FUNCTION "Gest Asse Y Foratrice" : VOID
TITLE =Gestione Asse Y Foratrice
AUTHOR : MassimoZ
FAMILY : NovaSrl
VERSION : 0.1

BEGIN
NETWORK
TITLE ======== PACO 1 =======



NETWORK
TITLE =INS./DISIN.1
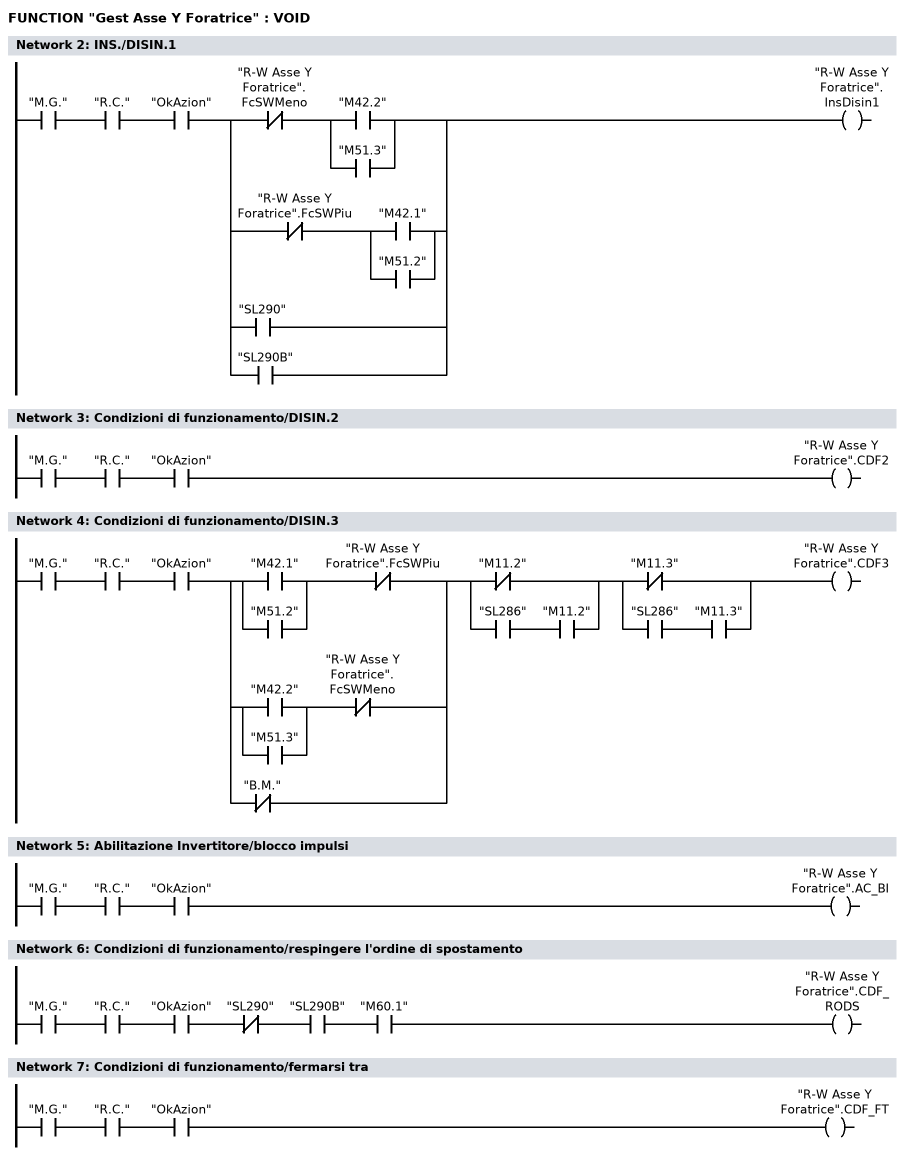
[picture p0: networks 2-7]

      U     "M.G.";
      U     "R.C.";
      U     "OkAzion";
      U(    ;
      UN    "R-W Asse Y Foratrice".FcSWMeno;
      U(    ;
      O     "M42.2";
      O     "M51.3";
      )     ;
      O     ;
      UN    "R-W Asse Y Foratrice".FcSWPiu;
      U(    ;
      O     "M42.1";
      O     "M51.2";
      )     ;
      O     "SL290";
      O     "SL290B";
      )     ;
      =     "R-W Asse Y Foratrice".InsDisin1;
NETWORK
TITLE =Condizioni di funzionamento/DISIN.2

      U     "M.G.";
      U     "R.C.";
      U     "OkAzion";
      =     "R-W Asse Y Foratrice".CDF2;
NETWORK
TITLE =Condizioni di funzionamento/DISIN.3

      U     "M.G.";
      U     "R.C.";
      U     "OkAzion";
      U(    ;
      U(    ;
      O     "M42.1";
      O     "M51.2";
      )     ;
      UN    "R-W Asse Y Foratrice".FcSWPiu;
      O     ;
      U(    ;
      O     "M42.2";
      O     "M51.3";
      )     ;
      UN    "R-W Asse Y Foratrice".FcSWMeno;
      ON    "B.M.";
      )     ;
      U(    ;
      ON    "M11.2";
      O     ;
      U     "SL286";
      U     "M11.2";
      )     ;
      U(    ;
      ON    "M11.3";
      O     ;
      U     "SL286";
      U     "M11.3";
      )     ;
      =     "R-W Asse Y Foratrice".CDF3;
NETWORK
TITLE =Abilitazione Invertitore/blocco impulsi

      U     "M.G.";
      U     "R.C.";
      U     "OkAzion";
      =     "R-W Asse Y Foratrice".AC_BI;
NETWORK
TITLE =Condizioni di funzionamento/respingere l'ordine di spostamento

      U     "M.G.";
      U     "R.C.";
      U     "OkAzion";
      UN    "SL290";
      U     "SL290B";
      U     "M60.1";
      =     "R-W Asse Y Foratrice".CDF_RODS;
NETWORK
TITLE =Condizioni di funzionamento/fermarsi tra

      U     "M.G.";
      U     "R.C.";
      U     "OkAzion";
      =     "R-W Asse Y Foratrice".CDF_FT;
NETWORK
TITLE =Attivare l'oridine di spostamento

      U(    ;
      U(    ;
      O     "M62.0";
      O     "M64.7";
      O     "M66.7";
      O     "M68.7";
      O     "M70.7";
      O     "M72.7";
      O     "M74.7";
      O     "M76.7";
      O     "M64.2";
      O     "M66.2";
      O     "M68.2";
      O     "M70.2";
      O     "M72.2";
      O     "M74.2";
      O     "M76.2";
      )     ;
      UN    "SL290";
      U     "SL290B";
      L     S5T#100MS;
      SE    T     12;
      NOP   0;
      NOP   0;
      NOP   0;
      U     T     12;
      )     ;
      FP    "FronteM251.2";
      =     "R-W Asse Y Foratrice".ALDS;
NETWORK
TITLE =Reset memoria guasti
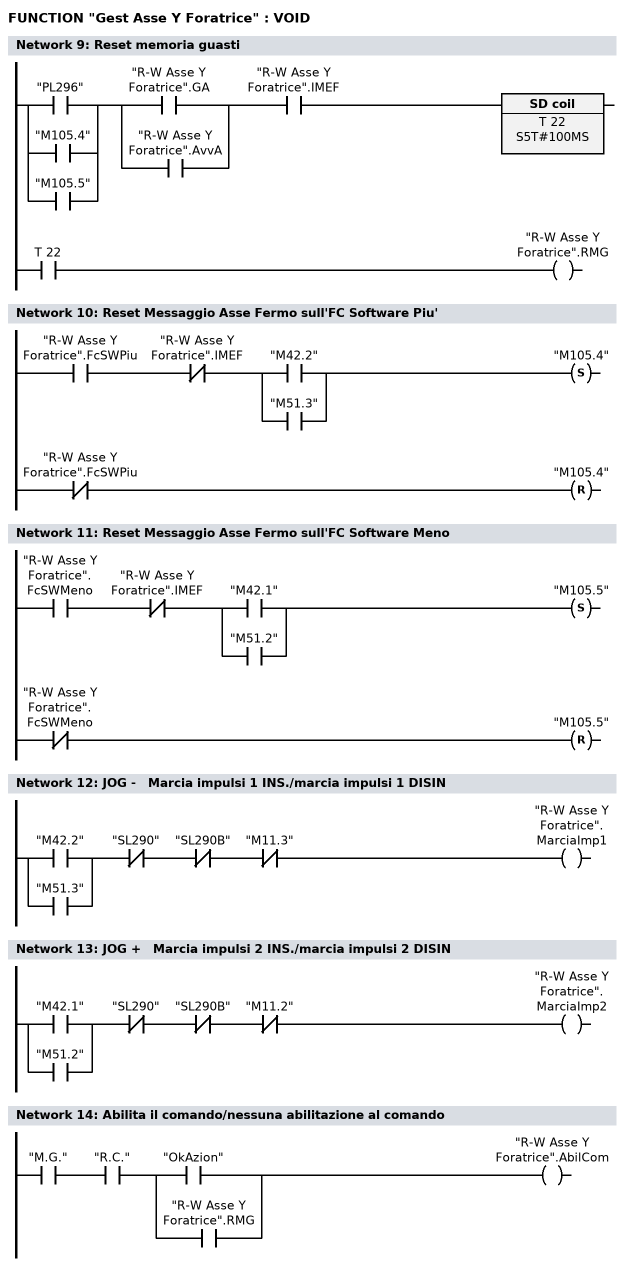
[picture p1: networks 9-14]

      U(    ;
      O     "PL296";
      O     "M105.4";
      O     "M105.5";
      )     ;
      U(    ;
      O     "R-W Asse Y Foratrice".GA;
      O     "R-W Asse Y Foratrice".AvvA;
      )     ;
      U     "R-W Asse Y Foratrice".IMEF;
      L     S5T#100MS;
      SE    T     22;
      NOP   0;
      NOP   0;
      NOP   0;
      U     T     22;
      =     "R-W Asse Y Foratrice".RMG;
NETWORK
TITLE =Reset Messaggio Asse Fermo sull'FC Software Piu'

      U     "R-W Asse Y Foratrice".FcSWPiu;
      UN    "R-W Asse Y Foratrice".IMEF;
      U(    ;
      O     "M42.2";
      O     "M51.3";
      )     ;
      S     "M105.4";
      UN    "R-W Asse Y Foratrice".FcSWPiu;
      R     "M105.4";
      NOP   0;
NETWORK
TITLE =Reset Messaggio Asse Fermo sull'FC Software Meno

      U     "R-W Asse Y Foratrice".FcSWMeno;
      UN    "R-W Asse Y Foratrice".IMEF;
      U(    ;
      O     "M42.1";
      O     "M51.2";
      )     ;
      S     "M105.5";
      UN    "R-W Asse Y Foratrice".FcSWMeno;
      R     "M105.5";
      NOP   0;
NETWORK
TITLE =JOG -   Marcia impulsi 1 INS./marcia impulsi 1 DISIN

      U(    ;
      O     "M42.2";
      O     "M51.3";
      )     ;
      UN    "SL290";
      UN    "SL290B";
      UN    "M11.3";
      =     "R-W Asse Y Foratrice".MarciaImp1;
NETWORK
TITLE =JOG +   Marcia impulsi 2 INS./marcia impulsi 2 DISIN

      U(    ;
      O     "M42.1";
      O     "M51.2";
      )     ;
      UN    "SL290";
      UN    "SL290B";
      UN    "M11.2";
      =     "R-W Asse Y Foratrice".MarciaImp2;
NETWORK
TITLE =Abilita il comando/nessuna abilitazione al comando

      U     "M.G.";
      U     "R.C.";
      U(    ;
      O     "OkAzion";
      O     "R-W Asse Y Foratrice".RMG;
      )     ;
      =     "R-W Asse Y Foratrice".AbilCom;
NETWORK
TITLE =Com Aut Apertura Pinza Foratrice per Ref Point

      U(    ;
      U     "SL290";
      UN    "SL290B";
      U     "PL292";
      S     "M105.6";
      U(    ;
      ON    "M.G.";
      ON    "SL290";
      O     "M11.2";
      O     "M11.3";
      )     ;
      R     "M105.6";
      U     "M105.6";
      )     ;
      L     "Scambio dati OP".TempApePinzaFor;
      SE    "T6";
      NOP   0;
      NOP   0;
      NOP   0;
      NOP   0;
NETWORK
TITLE =Avvio a riferirsi/interruzione del riferirsi
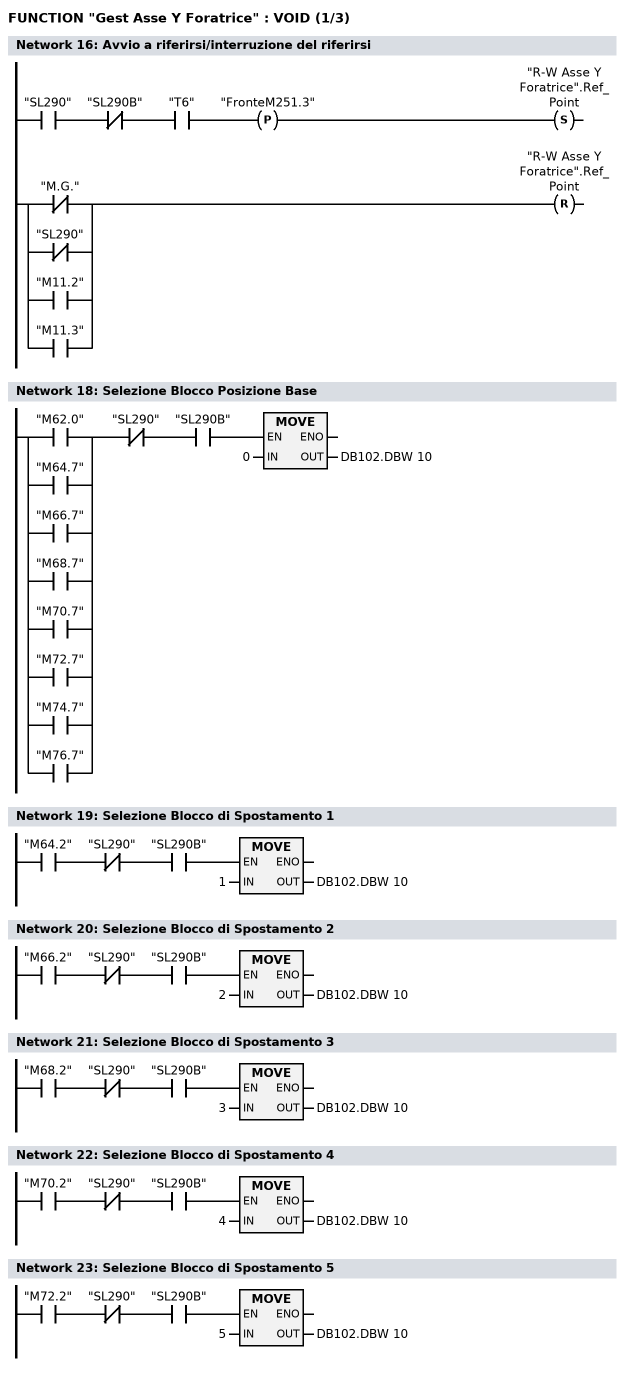
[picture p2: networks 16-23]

      U     "SL290";
      UN    "SL290B";
      U     "T6";
      FP    "FronteM251.3";
      S     "R-W Asse Y Foratrice".Ref_Point;
      U(    ;
      ON    "M.G.";
      ON    "SL290";
      O     "M11.2";
      O     "M11.3";
      )     ;
      R     "R-W Asse Y Foratrice".Ref_Point;
      NOP   0;
NETWORK
TITLE ======== SCELTA BLOCCO =======

NETWORK
TITLE =Selezione Blocco Posizione Base

      U(    ;
      O     "M62.0";
      O     "M64.7";
      O     "M66.7";
      O     "M68.7";
      O     "M70.7";
      O     "M72.7";
      O     "M74.7";
      O     "M76.7";
      )     ;
      UN    "SL290";
      U     "SL290B";
      SPBNB _001;
      L     0;
      T     DB102.DBW   10;
_001: NOP   0;
NETWORK
TITLE =Selezione Blocco di Spostamento 1

      U     "M64.2";
      UN    "SL290";
      U     "SL290B";
      SPBNB _002;
      L     1;
      T     DB102.DBW   10;
_002: NOP   0;
NETWORK
TITLE =Selezione Blocco di Spostamento 2

      U     "M66.2";
      UN    "SL290";
      U     "SL290B";
      SPBNB _003;
      L     2;
      T     DB102.DBW   10;
_003: NOP   0;
NETWORK
TITLE =Selezione Blocco di Spostamento 3

      U     "M68.2";
      UN    "SL290";
      U     "SL290B";
      SPBNB _004;
      L     3;
      T     DB102.DBW   10;
_004: NOP   0;
NETWORK
TITLE =Selezione Blocco di Spostamento 4

      U     "M70.2";
      UN    "SL290";
      U     "SL290B";
      SPBNB _005;
      L     4;
      T     DB102.DBW   10;
_005: NOP   0;
NETWORK
TITLE =Selezione Blocco di Spostamento 5

      U     "M72.2";
      UN    "SL290";
      U     "SL290B";
      SPBNB _006;
      L     5;
      T     DB102.DBW   10;
_006: NOP   0;
NETWORK
TITLE =Selezione Blocco di Spostamento 6
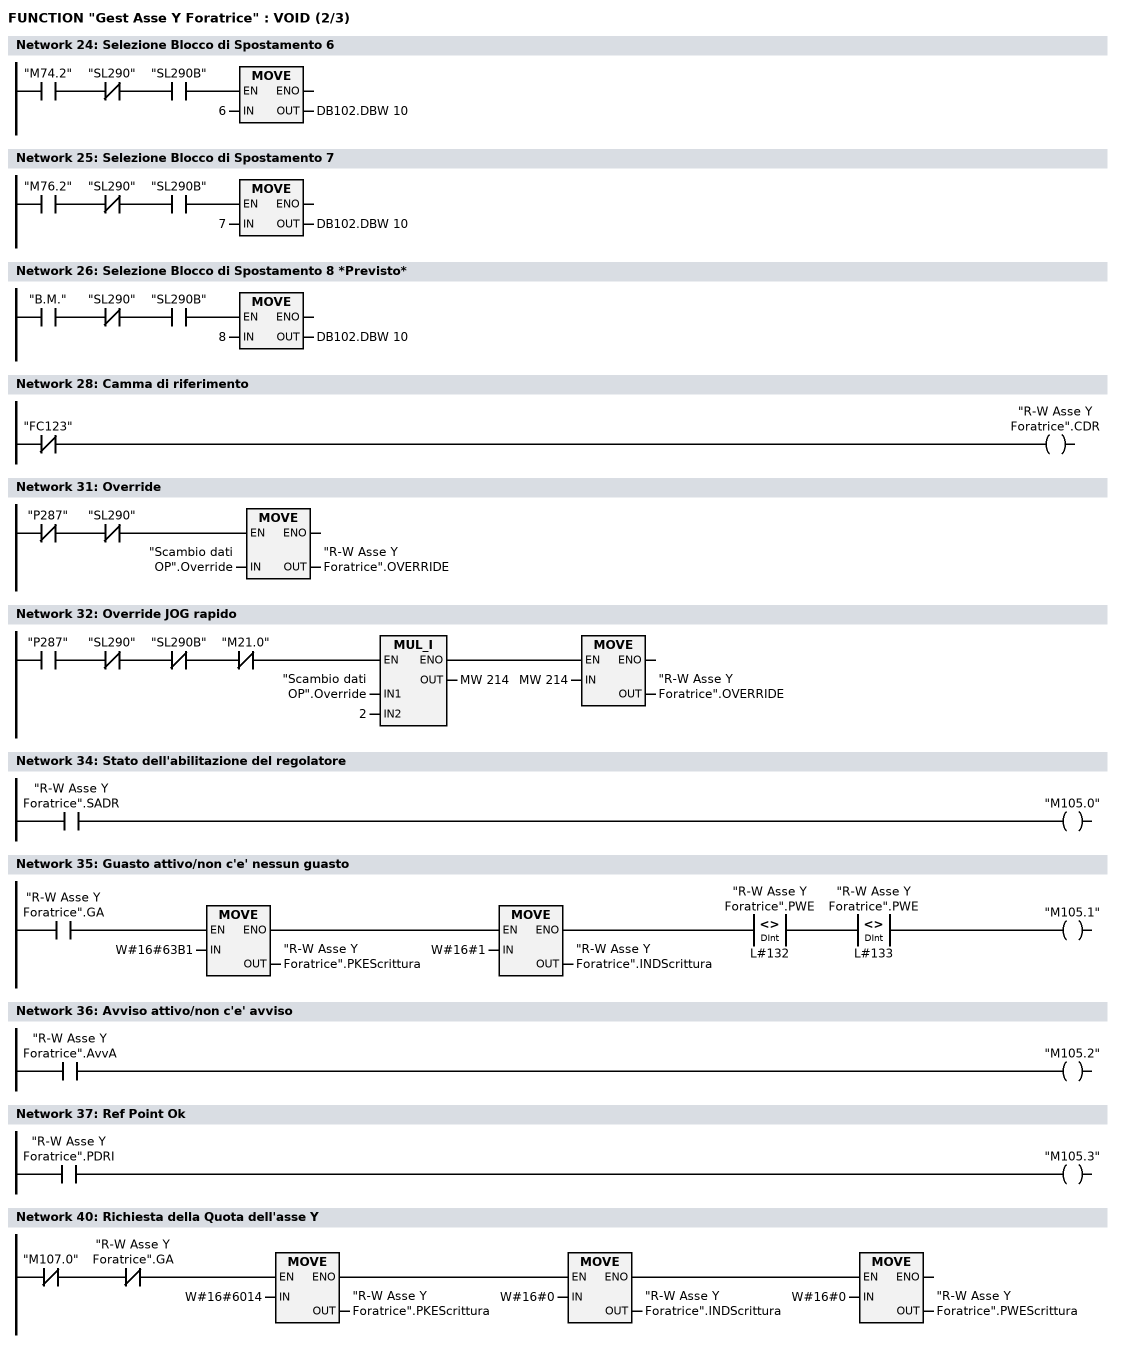
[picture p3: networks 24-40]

      U     "M74.2";
      UN    "SL290";
      U     "SL290B";
      SPBNB _007;
      L     6;
      T     DB102.DBW   10;
_007: NOP   0;
NETWORK
TITLE =Selezione Blocco di Spostamento 7

      U     "M76.2";
      UN    "SL290";
      U     "SL290B";
      SPBNB _008;
      L     7;
      T     DB102.DBW   10;
_008: NOP   0;
NETWORK
TITLE =Selezione Blocco di Spostamento 8 *Previsto*

      U     "B.M.";
      UN    "SL290";
      U     "SL290B";
      SPBNB _009;
      L     8;
      T     DB102.DBW   10;
_009: NOP   0;
NETWORK
TITLE ======== POS PACO =======



NETWORK
TITLE =Camma di riferimento

      UN    "FC123";
      =     "R-W Asse Y Foratrice".CDR;
NETWORK
TITLE ======== PACO 2 ======= ( previsto )



NETWORK
TITLE ======== OVERRIDE ======



NETWORK
TITLE =Override

      UN    "P287";
      UN    "SL290";
      SPBNB _00a;
      L     "Scambio dati OP".Override;
      T     "R-W Asse Y Foratrice".OVERRIDE;
_00a: NOP   0;
NETWORK
TITLE =Override JOG rapido

      U(    ;
      U     "P287";
      UN    "SL290";
      UN    "SL290B";
      UN    "M21.0";
      SPBNB _00b;
      L     "Scambio dati OP".Override;
      L     2;
      *I    ;
      T     MW   214;
      UN    OV;
      SAVE  ;
      CLR   ;
_00b: U     BIE;
      )     ;
      SPBNB _00c;
      L     MW   214;
      T     "R-W Asse Y Foratrice".OVERRIDE;
_00c: NOP   0;
NETWORK
TITLE ======== PAST 1 =======



NETWORK
TITLE =Stato dell'abilitazione del regolatore

      U     "R-W Asse Y Foratrice".SADR;
      =     "M105.0";
NETWORK
TITLE =Guasto attivo/non c'e' nessun guasto

      U(    ;
      U(    ;
      U     "R-W Asse Y Foratrice".GA;
      SPBNB _00d;
      L     W#16#63B1;
      T     "R-W Asse Y Foratrice".PKEScrittura;
      SET   ;
      SAVE  ;
      CLR   ;
_00d: U     BIE;
      )     ;
      SPBNB _00e;
      L     W#16#1;
      T     "R-W Asse Y Foratrice".INDScrittura;
      SET   ;
      SAVE  ;
      CLR   ;
_00e: U     BIE;
      )     ;
      U(    ;
      L     "R-W Asse Y Foratrice".PWE;
      L     L#132;
      <>D   ;
      )     ;
      U(    ;
      L     "R-W Asse Y Foratrice".PWE;
      L     L#133;
      <>D   ;
      )     ;
      =     "M105.1";
NETWORK
TITLE =Avviso attivo/non c'e' avviso

      U     "R-W Asse Y Foratrice".AvvA;
      =     "M105.2";
NETWORK
TITLE =Ref Point Ok

      U     "R-W Asse Y Foratrice".PDRI;
      =     "M105.3";
NETWORK
TITLE ======== POS PAST =======



NETWORK
TITLE ======== Lettura Quote =======



NETWORK
TITLE =Richiesta della Quota dell'asse Y

      U(    ;
      U(    ;
      UN    "M107.0";
      UN    "R-W Asse Y Foratrice".GA;
      SPBNB _00f;
      L     W#16#6014;
      T     "R-W Asse Y Foratrice".PKEScrittura;
      SET   ;
      SAVE  ;
      CLR   ;
_00f: U     BIE;
      )     ;
      SPBNB _010;
      L     W#16#0;
      T     "R-W Asse Y Foratrice".INDScrittura;
      SET   ;
      SAVE  ;
      CLR   ;
_010: U     BIE;
      )     ;
      SPBNB _011;
      L     W#16#0;
      T     "R-W Asse Y Foratrice".PWEScrittura;
_011: NOP   0;
NETWORK
TITLE =Lettura Quota Asse Y
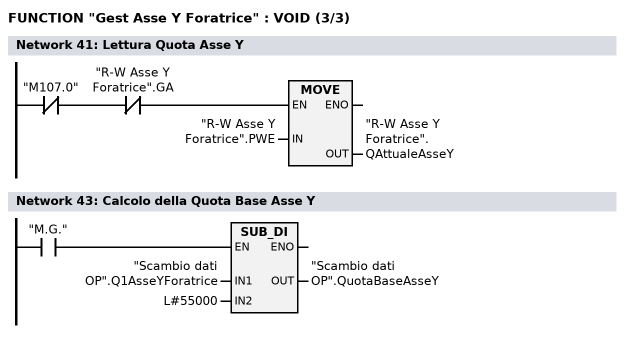
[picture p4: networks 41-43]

      UN    "M107.0";
      UN    "R-W Asse Y Foratrice".GA;
      SPBNB _012;
      L     "R-W Asse Y Foratrice".PWE;
      T     "R-W Asse Y Foratrice".QAttualeAsseY;
_012: NOP   0;
NETWORK
TITLE ======== Caricamento quote sui Blocchi di Spostamento =======



NETWORK
TITLE =Calcolo della Quota Base Asse Y

      U     "M.G.";
      SPBNB _013;
      L     "Scambio dati OP".Q1AsseYForatrice;
      L     L#55000;
      -D    ;
      T     "Scambio dati OP".QuotaBaseAsseY;
_013: NOP   0;
NETWORK
TITLE =Caricamento Primo Posizionamento

      UN    "SL290";
      UN    "SL290B";
      U     "Area Interfaccia OP  PLC".TDT;
      O     "M107.0";
      O(    ;
      U     "M.G.";
      FP    "FronteM252.6";
      )     ;
      =     L      0.0;
      U(    ;
      U(    ;
      U     L      0.0;
      UN    M    107.1;
      SPBNB _014;
      L     W#16#8051;
      T     "R-W Asse Y Foratrice".PKEScrittura;
      SET   ;
      SAVE  ;
      CLR   ;
_014: U     BIE;
      )     ;
      SPBNB _015;
      L     W#16#1;
      T     "R-W Asse Y Foratrice".INDScrittura;
      SET   ;
      SAVE  ;
      CLR   ;
_015: U     BIE;
      )     ;
      SPBNB _016;
      L     "Scambio dati OP".Q1AsseYForatrice;
      T     "R-W Asse Y Foratrice".PWEScrittura;
_016: NOP   0;
      U     L      0.0;
      BLD   102;
      S     "M107.0";
NETWORK
TITLE =Confronto Primo Posizionamento caricato nel 611U
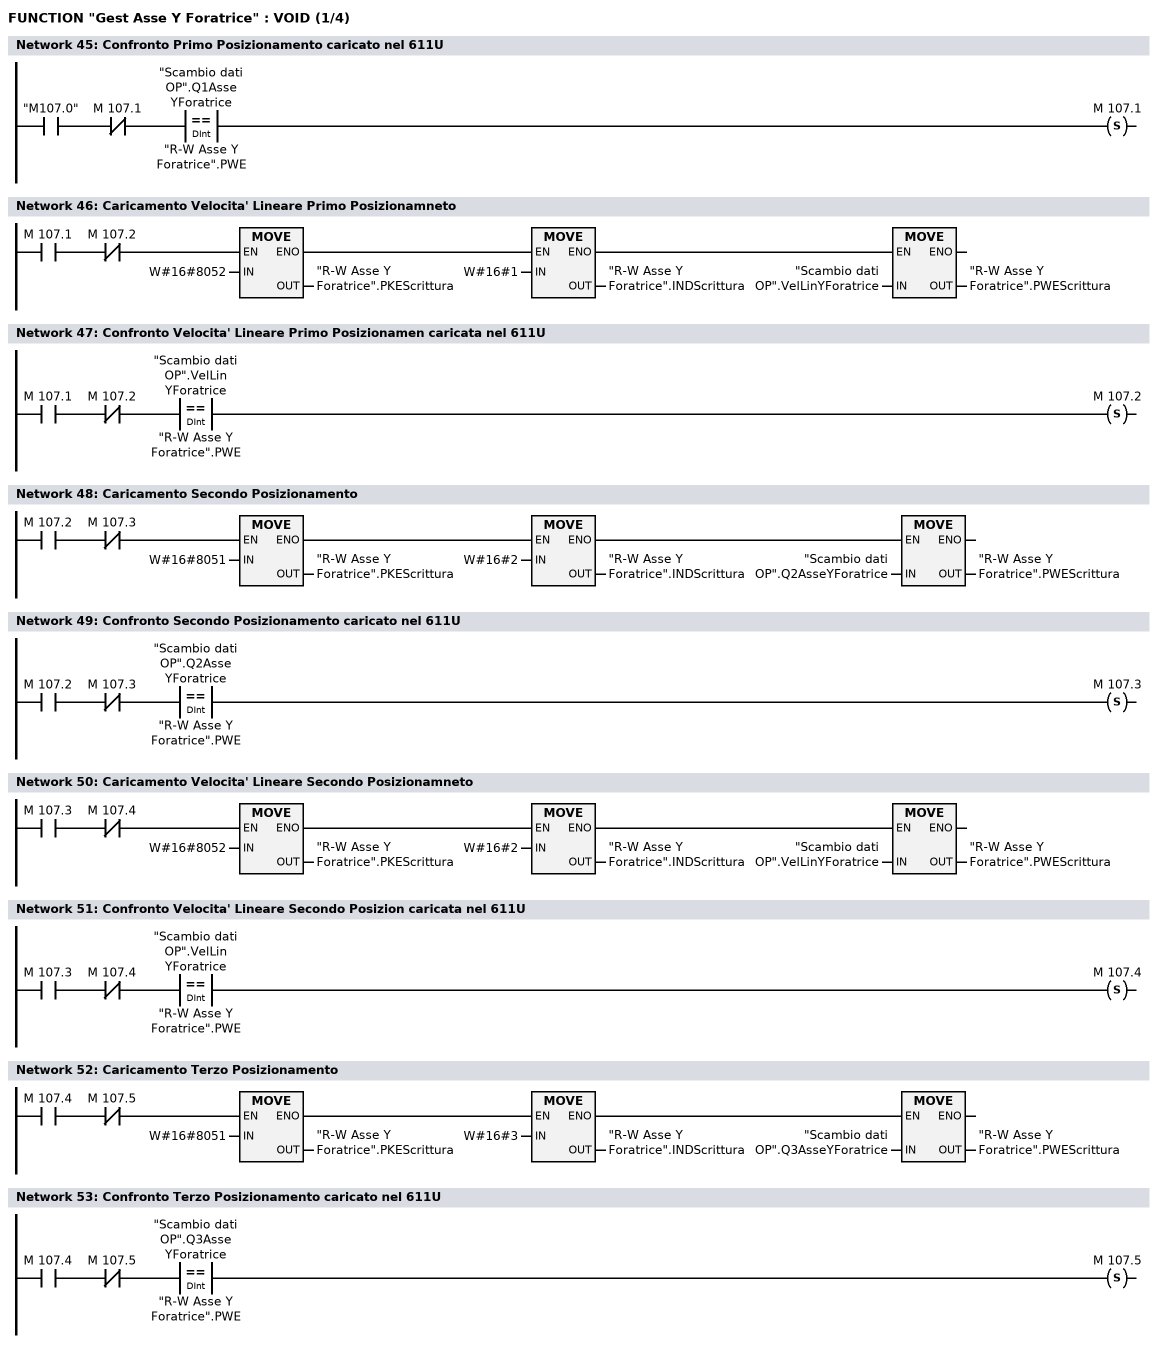
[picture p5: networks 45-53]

      U     "M107.0";
      UN    M    107.1;
      U(    ;
      L     "Scambio dati OP".Q1AsseYForatrice;
      L     "R-W Asse Y Foratrice".PWE;
      ==D   ;
      )     ;
      S     M    107.1;
NETWORK
TITLE =Caricamento Velocita' Lineare Primo Posizionamneto

      U(    ;
      U(    ;
      U     M    107.1;
      UN    M    107.2;
      SPBNB _017;
      L     W#16#8052;
      T     "R-W Asse Y Foratrice".PKEScrittura;
      SET   ;
      SAVE  ;
      CLR   ;
_017: U     BIE;
      )     ;
      SPBNB _018;
      L     W#16#1;
      T     "R-W Asse Y Foratrice".INDScrittura;
      SET   ;
      SAVE  ;
      CLR   ;
_018: U     BIE;
      )     ;
      SPBNB _019;
      L     "Scambio dati OP".VelLinYForatrice;
      T     "R-W Asse Y Foratrice".PWEScrittura;
_019: NOP   0;
NETWORK
TITLE =Confronto Velocita' Lineare Primo Posizionamen caricata nel 611U

      U     M    107.1;
      UN    M    107.2;
      U(    ;
      L     "Scambio dati OP".VelLinYForatrice;
      L     "R-W Asse Y Foratrice".PWE;
      ==D   ;
      )     ;
      S     M    107.2;
NETWORK
TITLE =Caricamento Secondo Posizionamento

      U(    ;
      U(    ;
      U     M    107.2;
      UN    M    107.3;
      SPBNB _01a;
      L     W#16#8051;
      T     "R-W Asse Y Foratrice".PKEScrittura;
      SET   ;
      SAVE  ;
      CLR   ;
_01a: U     BIE;
      )     ;
      SPBNB _01b;
      L     W#16#2;
      T     "R-W Asse Y Foratrice".INDScrittura;
      SET   ;
      SAVE  ;
      CLR   ;
_01b: U     BIE;
      )     ;
      SPBNB _01c;
      L     "Scambio dati OP".Q2AsseYForatrice;
      T     "R-W Asse Y Foratrice".PWEScrittura;
_01c: NOP   0;
NETWORK
TITLE =Confronto Secondo Posizionamento caricato nel 611U

      U     M    107.2;
      UN    M    107.3;
      U(    ;
      L     "Scambio dati OP".Q2AsseYForatrice;
      L     "R-W Asse Y Foratrice".PWE;
      ==D   ;
      )     ;
      S     M    107.3;
NETWORK
TITLE =Caricamento Velocita' Lineare Secondo Posizionamneto

      U(    ;
      U(    ;
      U     M    107.3;
      UN    M    107.4;
      SPBNB _01d;
      L     W#16#8052;
      T     "R-W Asse Y Foratrice".PKEScrittura;
      SET   ;
      SAVE  ;
      CLR   ;
_01d: U     BIE;
      )     ;
      SPBNB _01e;
      L     W#16#2;
      T     "R-W Asse Y Foratrice".INDScrittura;
      SET   ;
      SAVE  ;
      CLR   ;
_01e: U     BIE;
      )     ;
      SPBNB _01f;
      L     "Scambio dati OP".VelLinYForatrice;
      T     "R-W Asse Y Foratrice".PWEScrittura;
_01f: NOP   0;
NETWORK
TITLE =Confronto Velocita' Lineare Secondo Posizion caricata nel 611U

      U     M    107.3;
      UN    M    107.4;
      U(    ;
      L     "Scambio dati OP".VelLinYForatrice;
      L     "R-W Asse Y Foratrice".PWE;
      ==D   ;
      )     ;
      S     M    107.4;
NETWORK
TITLE =Caricamento Terzo Posizionamento

      U(    ;
      U(    ;
      U     M    107.4;
      UN    M    107.5;
      SPBNB _020;
      L     W#16#8051;
      T     "R-W Asse Y Foratrice".PKEScrittura;
      SET   ;
      SAVE  ;
      CLR   ;
_020: U     BIE;
      )     ;
      SPBNB _021;
      L     W#16#3;
      T     "R-W Asse Y Foratrice".INDScrittura;
      SET   ;
      SAVE  ;
      CLR   ;
_021: U     BIE;
      )     ;
      SPBNB _022;
      L     "Scambio dati OP".Q3AsseYForatrice;
      T     "R-W Asse Y Foratrice".PWEScrittura;
_022: NOP   0;
NETWORK
TITLE =Confronto Terzo Posizionamento caricato nel 611U

      U     M    107.4;
      UN    M    107.5;
      U(    ;
      L     "Scambio dati OP".Q3AsseYForatrice;
      L     "R-W Asse Y Foratrice".PWE;
      ==D   ;
      )     ;
      S     M    107.5;
NETWORK
TITLE =Caricamento Velocita' Lineare Terzo Posizionamento
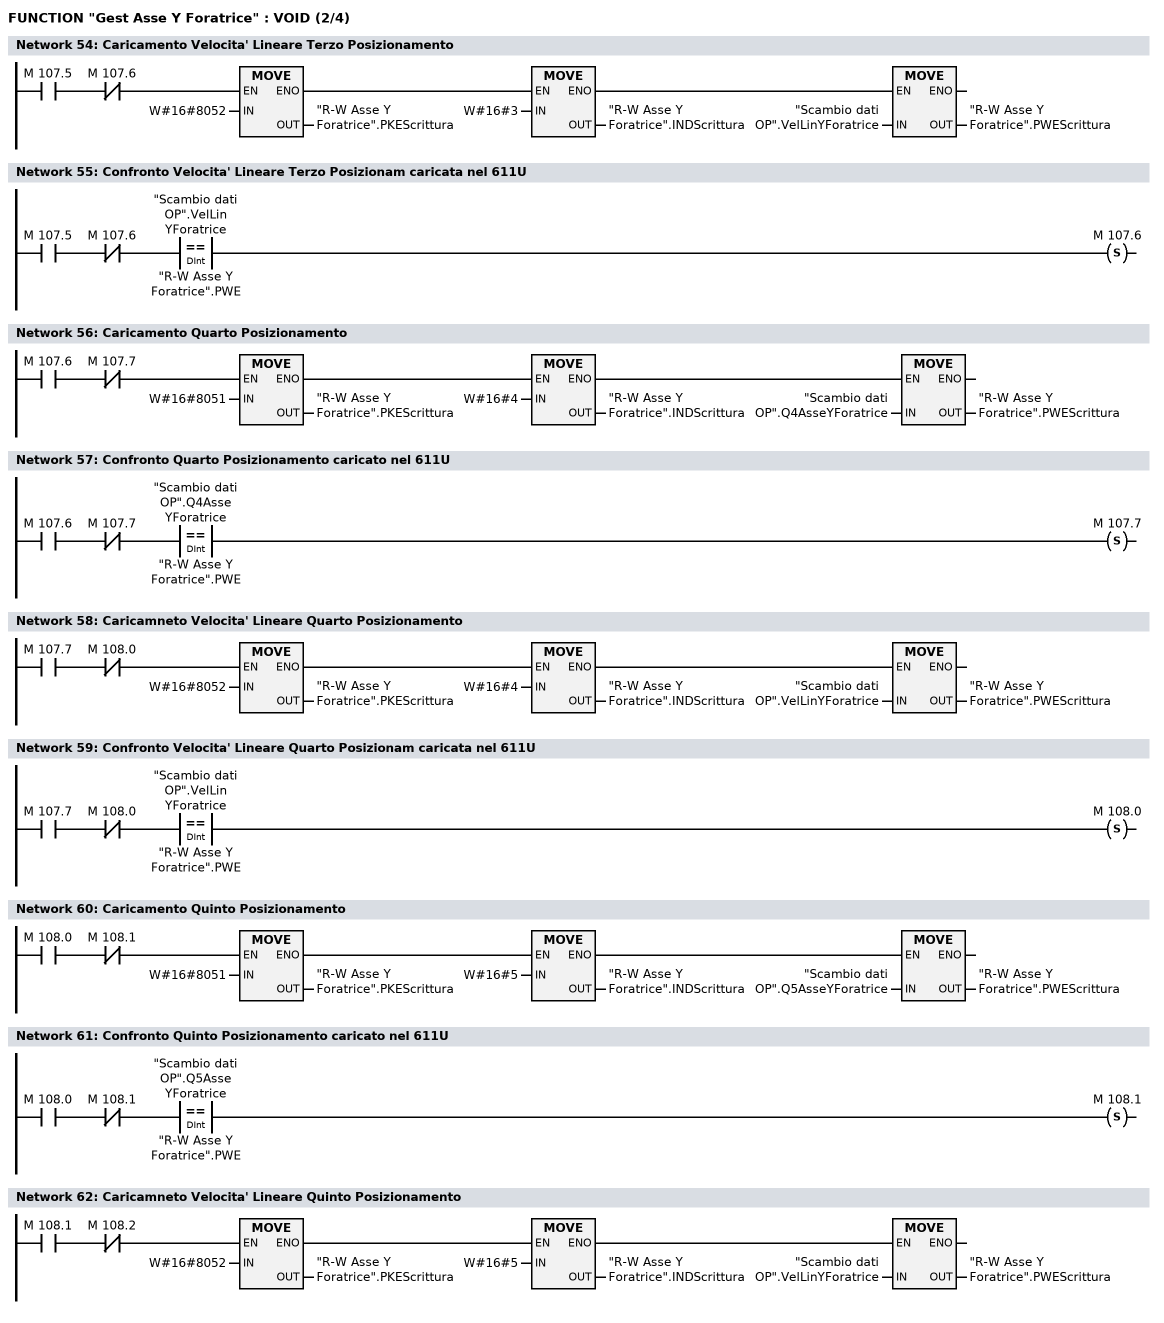
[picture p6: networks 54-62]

      U(    ;
      U(    ;
      U     M    107.5;
      UN    M    107.6;
      SPBNB _023;
      L     W#16#8052;
      T     "R-W Asse Y Foratrice".PKEScrittura;
      SET   ;
      SAVE  ;
      CLR   ;
_023: U     BIE;
      )     ;
      SPBNB _024;
      L     W#16#3;
      T     "R-W Asse Y Foratrice".INDScrittura;
      SET   ;
      SAVE  ;
      CLR   ;
_024: U     BIE;
      )     ;
      SPBNB _025;
      L     "Scambio dati OP".VelLinYForatrice;
      T     "R-W Asse Y Foratrice".PWEScrittura;
_025: NOP   0;
NETWORK
TITLE =Confronto Velocita' Lineare Terzo Posizionam caricata nel 611U

      U     M    107.5;
      UN    M    107.6;
      U(    ;
      L     "Scambio dati OP".VelLinYForatrice;
      L     "R-W Asse Y Foratrice".PWE;
      ==D   ;
      )     ;
      S     M    107.6;
NETWORK
TITLE =Caricamento Quarto Posizionamento

      U(    ;
      U(    ;
      U     M    107.6;
      UN    M    107.7;
      SPBNB _026;
      L     W#16#8051;
      T     "R-W Asse Y Foratrice".PKEScrittura;
      SET   ;
      SAVE  ;
      CLR   ;
_026: U     BIE;
      )     ;
      SPBNB _027;
      L     W#16#4;
      T     "R-W Asse Y Foratrice".INDScrittura;
      SET   ;
      SAVE  ;
      CLR   ;
_027: U     BIE;
      )     ;
      SPBNB _028;
      L     "Scambio dati OP".Q4AsseYForatrice;
      T     "R-W Asse Y Foratrice".PWEScrittura;
_028: NOP   0;
NETWORK
TITLE =Confronto Quarto Posizionamento caricato nel 611U

      U     M    107.6;
      UN    M    107.7;
      U(    ;
      L     "Scambio dati OP".Q4AsseYForatrice;
      L     "R-W Asse Y Foratrice".PWE;
      ==D   ;
      )     ;
      S     M    107.7;
NETWORK
TITLE =Caricamneto Velocita' Lineare Quarto Posizionamento

      U(    ;
      U(    ;
      U     M    107.7;
      UN    M    108.0;
      SPBNB _029;
      L     W#16#8052;
      T     "R-W Asse Y Foratrice".PKEScrittura;
      SET   ;
      SAVE  ;
      CLR   ;
_029: U     BIE;
      )     ;
      SPBNB _02a;
      L     W#16#4;
      T     "R-W Asse Y Foratrice".INDScrittura;
      SET   ;
      SAVE  ;
      CLR   ;
_02a: U     BIE;
      )     ;
      SPBNB _02b;
      L     "Scambio dati OP".VelLinYForatrice;
      T     "R-W Asse Y Foratrice".PWEScrittura;
_02b: NOP   0;
NETWORK
TITLE =Confronto Velocita' Lineare Quarto Posizionam caricata nel 611U

      U     M    107.7;
      UN    M    108.0;
      U(    ;
      L     "Scambio dati OP".VelLinYForatrice;
      L     "R-W Asse Y Foratrice".PWE;
      ==D   ;
      )     ;
      S     M    108.0;
NETWORK
TITLE =Caricamento Quinto Posizionamento

      U(    ;
      U(    ;
      U     M    108.0;
      UN    M    108.1;
      SPBNB _02c;
      L     W#16#8051;
      T     "R-W Asse Y Foratrice".PKEScrittura;
      SET   ;
      SAVE  ;
      CLR   ;
_02c: U     BIE;
      )     ;
      SPBNB _02d;
      L     W#16#5;
      T     "R-W Asse Y Foratrice".INDScrittura;
      SET   ;
      SAVE  ;
      CLR   ;
_02d: U     BIE;
      )     ;
      SPBNB _02e;
      L     "Scambio dati OP".Q5AsseYForatrice;
      T     "R-W Asse Y Foratrice".PWEScrittura;
_02e: NOP   0;
NETWORK
TITLE =Confronto Quinto Posizionamento caricato nel 611U

      U     M    108.0;
      UN    M    108.1;
      U(    ;
      L     "Scambio dati OP".Q5AsseYForatrice;
      L     "R-W Asse Y Foratrice".PWE;
      ==D   ;
      )     ;
      S     M    108.1;
NETWORK
TITLE =Caricamneto Velocita' Lineare Quinto Posizionamento

      U(    ;
      U(    ;
      U     M    108.1;
      UN    M    108.2;
      SPBNB _02f;
      L     W#16#8052;
      T     "R-W Asse Y Foratrice".PKEScrittura;
      SET   ;
      SAVE  ;
      CLR   ;
_02f: U     BIE;
      )     ;
      SPBNB _030;
      L     W#16#5;
      T     "R-W Asse Y Foratrice".INDScrittura;
      SET   ;
      SAVE  ;
      CLR   ;
_030: U     BIE;
      )     ;
      SPBNB _031;
      L     "Scambio dati OP".VelLinYForatrice;
      T     "R-W Asse Y Foratrice".PWEScrittura;
_031: NOP   0;
NETWORK
TITLE =Confronto Velocita' Lineare Quinto Posizionam caricata nel 611U
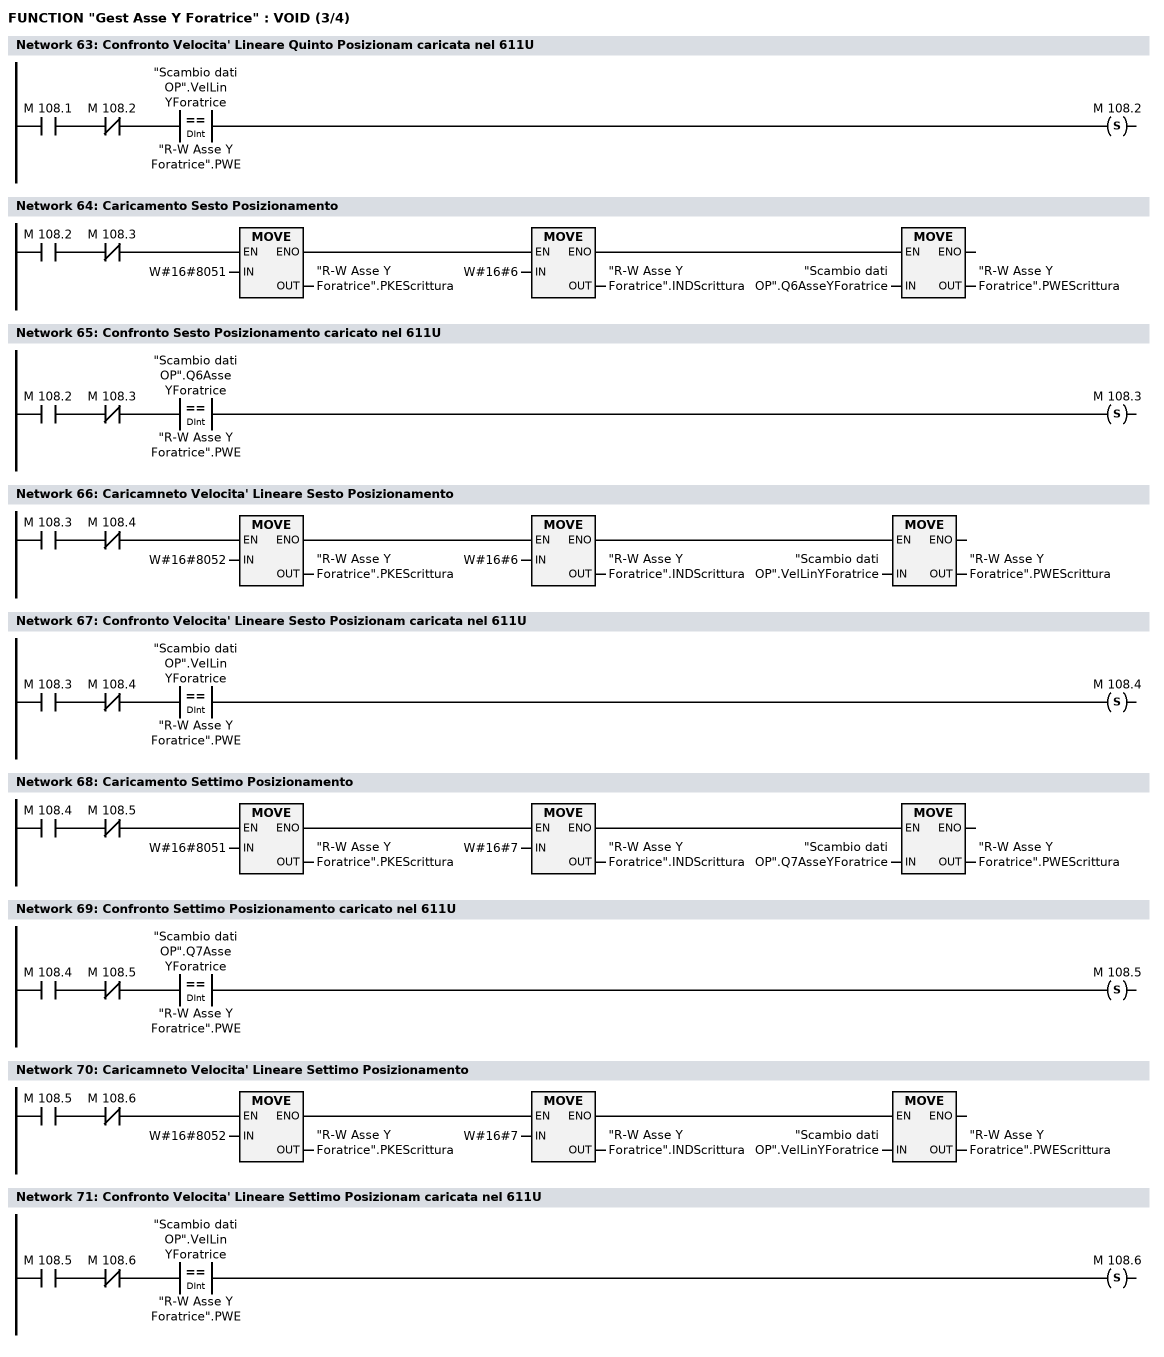
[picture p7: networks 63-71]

      U     M    108.1;
      UN    M    108.2;
      U(    ;
      L     "Scambio dati OP".VelLinYForatrice;
      L     "R-W Asse Y Foratrice".PWE;
      ==D   ;
      )     ;
      S     M    108.2;
NETWORK
TITLE =Caricamento Sesto Posizionamento

      U(    ;
      U(    ;
      U     M    108.2;
      UN    M    108.3;
      SPBNB _032;
      L     W#16#8051;
      T     "R-W Asse Y Foratrice".PKEScrittura;
      SET   ;
      SAVE  ;
      CLR   ;
_032: U     BIE;
      )     ;
      SPBNB _033;
      L     W#16#6;
      T     "R-W Asse Y Foratrice".INDScrittura;
      SET   ;
      SAVE  ;
      CLR   ;
_033: U     BIE;
      )     ;
      SPBNB _034;
      L     "Scambio dati OP".Q6AsseYForatrice;
      T     "R-W Asse Y Foratrice".PWEScrittura;
_034: NOP   0;
NETWORK
TITLE =Confronto Sesto Posizionamento caricato nel 611U

      U     M    108.2;
      UN    M    108.3;
      U(    ;
      L     "Scambio dati OP".Q6AsseYForatrice;
      L     "R-W Asse Y Foratrice".PWE;
      ==D   ;
      )     ;
      S     M    108.3;
NETWORK
TITLE =Caricamneto Velocita' Lineare Sesto Posizionamento

      U(    ;
      U(    ;
      U     M    108.3;
      UN    M    108.4;
      SPBNB _035;
      L     W#16#8052;
      T     "R-W Asse Y Foratrice".PKEScrittura;
      SET   ;
      SAVE  ;
      CLR   ;
_035: U     BIE;
      )     ;
      SPBNB _036;
      L     W#16#6;
      T     "R-W Asse Y Foratrice".INDScrittura;
      SET   ;
      SAVE  ;
      CLR   ;
_036: U     BIE;
      )     ;
      SPBNB _037;
      L     "Scambio dati OP".VelLinYForatrice;
      T     "R-W Asse Y Foratrice".PWEScrittura;
_037: NOP   0;
NETWORK
TITLE =Confronto Velocita' Lineare Sesto Posizionam caricata nel 611U

      U     M    108.3;
      UN    M    108.4;
      U(    ;
      L     "Scambio dati OP".VelLinYForatrice;
      L     "R-W Asse Y Foratrice".PWE;
      ==D   ;
      )     ;
      S     M    108.4;
NETWORK
TITLE =Caricamento Settimo Posizionamento

      U(    ;
      U(    ;
      U     M    108.4;
      UN    M    108.5;
      SPBNB _038;
      L     W#16#8051;
      T     "R-W Asse Y Foratrice".PKEScrittura;
      SET   ;
      SAVE  ;
      CLR   ;
_038: U     BIE;
      )     ;
      SPBNB _039;
      L     W#16#7;
      T     "R-W Asse Y Foratrice".INDScrittura;
      SET   ;
      SAVE  ;
      CLR   ;
_039: U     BIE;
      )     ;
      SPBNB _03a;
      L     "Scambio dati OP".Q7AsseYForatrice;
      T     "R-W Asse Y Foratrice".PWEScrittura;
_03a: NOP   0;
NETWORK
TITLE =Confronto Settimo Posizionamento caricato nel 611U

      U     M    108.4;
      UN    M    108.5;
      U(    ;
      L     "Scambio dati OP".Q7AsseYForatrice;
      L     "R-W Asse Y Foratrice".PWE;
      ==D   ;
      )     ;
      S     M    108.5;
NETWORK
TITLE =Caricamneto Velocita' Lineare Settimo Posizionamento

      U(    ;
      U(    ;
      U     M    108.5;
      UN    M    108.6;
      SPBNB _03b;
      L     W#16#8052;
      T     "R-W Asse Y Foratrice".PKEScrittura;
      SET   ;
      SAVE  ;
      CLR   ;
_03b: U     BIE;
      )     ;
      SPBNB _03c;
      L     W#16#7;
      T     "R-W Asse Y Foratrice".INDScrittura;
      SET   ;
      SAVE  ;
      CLR   ;
_03c: U     BIE;
      )     ;
      SPBNB _03d;
      L     "Scambio dati OP".VelLinYForatrice;
      T     "R-W Asse Y Foratrice".PWEScrittura;
_03d: NOP   0;
NETWORK
TITLE =Confronto Velocita' Lineare Settimo Posizionam caricata nel 611U

      U     M    108.5;
      UN    M    108.6;
      U(    ;
      L     "Scambio dati OP".VelLinYForatrice;
      L     "R-W Asse Y Foratrice".PWE;
      ==D   ;
      )     ;
      S     M    108.6;
NETWORK
TITLE =Caricamento Posizionamento Base
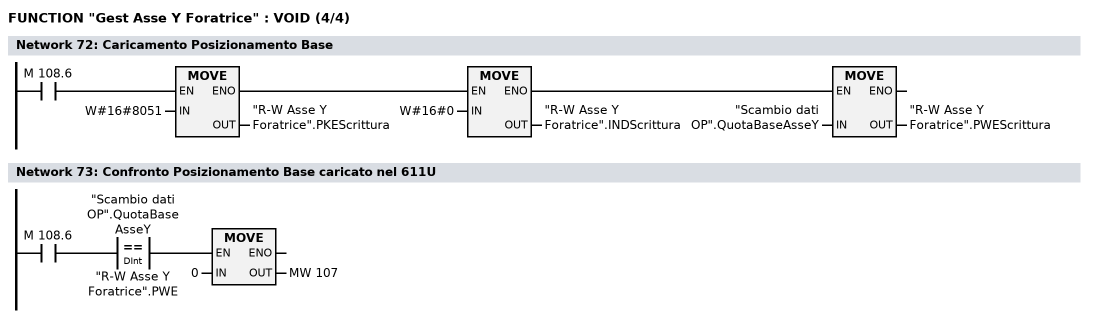
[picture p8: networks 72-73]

      U(    ;
      U(    ;
      U     M    108.6;
      SPBNB _03e;
      L     W#16#8051;
      T     "R-W Asse Y Foratrice".PKEScrittura;
      SET   ;
      SAVE  ;
      CLR   ;
_03e: U     BIE;
      )     ;
      SPBNB _03f;
      L     W#16#0;
      T     "R-W Asse Y Foratrice".INDScrittura;
      SET   ;
      SAVE  ;
      CLR   ;
_03f: U     BIE;
      )     ;
      SPBNB _040;
      L     "Scambio dati OP".QuotaBaseAsseY;
      T     "R-W Asse Y Foratrice".PWEScrittura;
_040: NOP   0;
NETWORK
TITLE =Confronto Posizionamento Base caricato nel 611U

      U     M    108.6;
      U(    ;
      L     "Scambio dati OP".QuotaBaseAsseY;
      L     "R-W Asse Y Foratrice".PWE;
      ==D   ;
      )     ;
      SPBNB _041;
      L     0;
      T     MW   107;
_041: NOP   0;
END_FUNCTION

